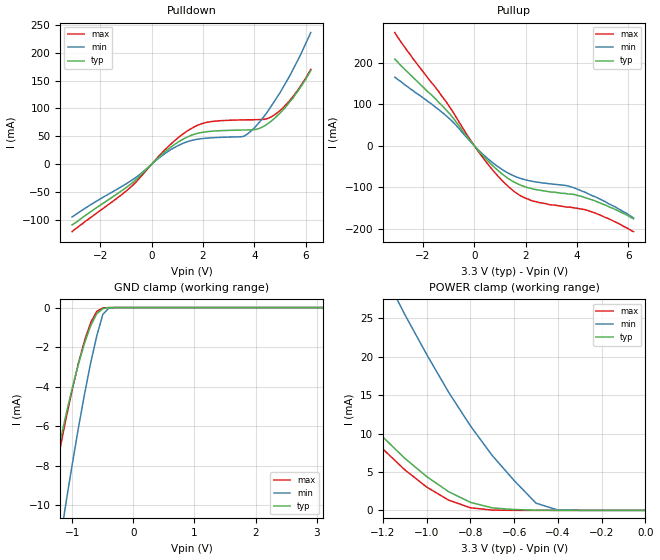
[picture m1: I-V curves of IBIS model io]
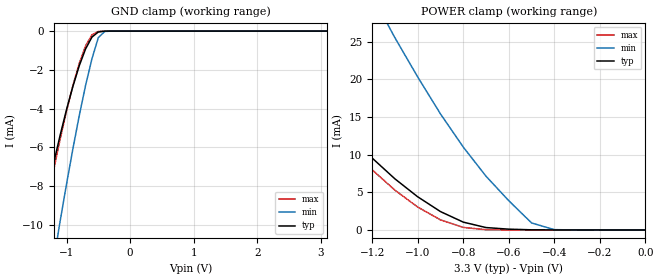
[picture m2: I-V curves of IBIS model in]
[IBIS Ver]   1.1
[File name]   m63733a.ibs
[File Rev]   1.0
[Date]   7/28/98
[Source]   This file originated at Motorola Fast SRAM.
[Notes]
 1. This I/O model good for MCM63733A 128Kx32 4Mb BurstRAM "F" and "P" versions (TQFP).
[Disclaimer]   Data is for modeling purposes only and is not guaranteed
[Component]   128Kx32 4Mb BurstRAM
[Manufacturer] Motorola
[Package]
|  RLC Data is subject to change after further study of package
|		typ		min		max
R_pkg		200m		150m		250m
L_pkg		5.5nH		4nH		7nH
C_pkg		2pF		1.5pF		2.5pF
[Pin]		signal_name	model_name	R_pin		L_pin		C_pin
1		NC		NC		NA		NA		NA
2		DCc		io		NA		NA		NA
3		DCc		io		NA		NA		NA
4		VDDQ		POWER		NA		NA		NA
5		VSS		GND		NA		NA		NA
6		DCc		io		NA		NA		NA
7		DCc		io		NA		NA		NA
8		DQc		io		NA		NA		NA
9		DQc		io		NA		NA		NA
10		VSS		GND		NA		NA		NA
11		VDDQ		POWER		NA		NA		NA
12		DQc		io		NA		NA		NA
13		DQc		io		NA		NA		NA
14		NC		NC		NA		NA		NA
15		VDD		POWER		NA		NA		NA
16		NC		NC		NA		NA		NA
17		VSS		GND		NA		NA		NA
18		DQd		io		NA		NA		NA
19		DQd	 	io		NA		NA		NA
20		VDDQ		POWER		NA		NA		NA
21		VSS		GND		NA		NA		NA
22		DQd		io		NA		NA		NA
23		DQd		io		NA		NA		NA
24		DQd		io		NA		NA		NA
25		DCd		io		NA		NA		NA
26		VSS		GND		NA		NA		NA
27		VDDQ		POWER		NA		NA		NA
28		DCd		io		NA		NA		NA
29		DCd		io		NA		NA		NA
30		NC		NC		NA		NA		NA
31		LBO#		NC		NA		NA		NA
32		SA		in		NA		NA		NA
33		SA		in		NA		NA		NA
34		SA		in		NA		NA		NA
35		SA		in		NA		NA		NA
36		SA1		in		NA		NA		NA
37		SA0		in		NA		NA		NA
38		NC		NC		NA		NA		NA
39		NC		NC		NA		NA		NA
40		VSS		GND		NA		NA		NA
41		VDD		POWER		NA		NA		NA
42		NC		NC		NA		NA		NA
43		NC		NC		NA		NA		NA
44		SA		in		NA		NA		NA
45		SA		in		NA		NA		NA
46		SA		in		NA		NA		NA
47		SA		in		NA		NA		NA
48		SA		in		NA		NA		NA
49		SA		in		NA		NA		NA
50		SA		in		NA		NA		NA
51		NC		NC		NA		NA		NA
52		DQa		io		NA		NA		NA
53		DQa		io		NA		NA		NA
54		VDDQ		POWER		NA		NA		NA
55		VSS		GND		NA		NA		NA
56		DQa		io		NA		NA		NA
57		DQa		io		NA		NA		NA
58		DQa		io		NA		NA		NA
59		DQa		io		NA		NA		NA
60		VSS		GND		NA		NA		NA
61		VDDQ		POWER		NA		NA		NA
62		DQa		io		NA		NA		NA
63		DQa		io		NA		NA		NA
64		ZZ		NC		NA		NA		NA
65		VDD		POWER		NA		NA		NA
66		NC		NC		NA		NA		NA
67		VSS		GND		NA		NA		NA
68		DQb		io		NA		NA		NA
69		DQb		io		NA		NA		NA
70		VDDQ		POWER		NA		NA		NA
71		VSS		GND		NA		NA		NA
72		DQb		io		NA		NA		NA
73		DQb		io		NA		NA		NA
74		DQb		io		NA		NA		NA
75		DQb		io		NA		NA		NA
76		VSS		GND		NA		NA		NA
77		VDDQ		POWER		NA		NA		NA
78		DQb		io		NA		NA		NA
79		DQb		io		NA		NA		NA
80		NC		NC		NA		NA		NA
81		SA		in		NA		NA		NA
82		SA		in		NA		NA		NA
83		ADV		in		NA		NA		NA
84		ADSP		in		NA		NA		NA
85		ADSC		in		NA		NA		NA
86		G#		in		NA		NA		NA
87		SW#		in		NA		NA		NA
88		SGW#		in		NA		NA		NA
89		K		in		NA		NA		NA
90		VSS		GND		NA		NA		NA
91		VDD		POWER		NA		NA		NA
92		SE3#		in		NA		NA		NA
93		SBA#		in		NA		NA		NA
94		SBB#		in		NA		NA		NA
95		SBC#		NC		NA		NA		NA
96		SBD#		NC		NA		NA		NA
97		SE2		in		NA		NA		NA
98		SE1#		in		NA		NA		NA
99		SA		in		NA		NA		NA
100		SA		in		NA		NA		NA
| Models and submodels in the file (2): io (I/O), in (Input)
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| BI-DIRECTIONAL I/O MODEL
[Model]   io
Model_type  I/O
Polarity   Non-Inverting
Enable   Active-Low
|signals  DQa, DQb, DQc, DQd
|Variable   typ   min   max
C_comp   7pF   NA   8pF
|Variable   typ   min   max
[Voltage range]   3.3   3.1  3.6
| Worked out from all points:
|   slope of the pulldown table from 0 to 0.495 V, typ, clamps not added: 23.3 ohm
|   slope of the pullup table from 0 to 0.495 V, typ, clamps not added: 14.4 ohm
|   GND clamp passes 1 mA (typ) near -0.71 V on its own axis
|   POWER clamp passes 1 mA (typ) near -0.79 V on its own axis
|Temp used   50C   100C   0C
|Variable   typ   min   max
|NOTE: All V/I tables should have at least 3 entries.
|   0.0 volts, 2*supply_voltage and -supply_voltage
[Pulldown]
|Volt	Typical		Minimum		Maximum
-3.1V     -109mA     -94.7mA    -121mA
-900mV    -38.8mA    -32.6mA    -44.6mA
500mV     21.4mA     18.4mA     25mA
1.4V      48.9mA     40.4mA     59.8mA
2.2V      58.5mA     46.8mA     75.4mA
3.5V      61.2mA     49.2mA     79.3mA
3.8V      61.4mA     56.5mA     79.6mA
4.3V      66.3mA     81mA       80mA
4.6V      75.1mA     99.8mA     83.5mA
4.9V      87mA       121mA      92.3mA
5.4V      113mA      160mA      115mA
6.2V      168mA      236mA      170mA
[Pullup]
|Volt	Typical		Minimum		Maximum
-3.1V     208mA      165mA      272mA
-2.4V     165mA      133mA      210mA
-1.1V     86.2mA     72.2mA     106mA
-200mV    15.4mA     13.3mA     18.3mA
300mV     -21.4mA    -18.4mA    -25.8mA
900mV     -58.1mA    -49.2mA    -71.3mA
1.4V      -81.6mA    -68.2mA    -102mA
1.8V      -94.4mA    -78.2mA    -120mA
2.3V      -104mA     -85.6mA    -133mA
3.9V      -117mA     -101mA     -149mA
4.7V      -132mA     -122mA     -161mA
6.2V      -175mA     -173mA     -206mA
[GND_clamp]
|Volt	Typical		Minimum		Maximum
-3.1V     -45.8mA    -60.1mA    -49.3mA
-1.5V     -11.5mA    -18.1mA    -12.3mA
-1.4V     -9.83mA    -15.9mA    -10.5mA
-1.2V     -6.78mA    -11.8mA    -7.13mA
-1.1V     -5.37mA    -9.8mA     -5.57mA
-900mV    -2.86mA    -6.08mA    -2.81mA
-800mV    -1.79mA    -4.37mA    -1.67mA
-700mV    -918uA     -2.8mA     -759uA
-600mV    -310uA     -1.43mA    -192uA
-500mV    -48.2uA    -340uA     -17.7uA
-300mV    -165nA     -1.28uA    -19.6nA
3.1V      425pA      626pA      394pA
[POWER_clamp]
|Volt	Typical		Minimum		Maximum
-3.1V     105mA      173mA      110mA
-1.7V     27.7mA     62.5mA     26.7mA
-1.6V     23.6mA     55.8mA     22.4mA
-1.4V     16mA       43mA       14.5mA
-1.2V     9.54mA     31.1mA     7.98mA
-1.1V     6.78mA     25.5mA     5.28mA
-900mV    2.44mA     15.4mA     1.34mA
-800mV    1.04mA     11mA       338uA
-700mV    319uA      7.13mA     33.9uA
-500mV    20.9uA     933uA      150nA
-400mV    578nA      41.7uA     2.74nA
0V        469pA      626pA      504pA
[Ramp]
|Variable   typ   min	max
dV/dt_r  1.50/0.33n	NA	NA
dV/dt_f  1.29/0.13n	NA	NA
| STANDARD INPUT MODEL
[Model]   in
Model_type  Input
Polarity   Non-Inverting
|signals  ADSP#, ADSC#, ADV#, G#, K, SA, SBx#, SE1#, SE2, SE3#, SGW#, SW#
|Variable   typ   min   max
C_comp   4pF   NA   5pF
|Variable   typ   min   max
[Voltage range]   3.3   3.1  3.6
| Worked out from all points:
|   GND clamp passes 1 mA (typ) near -0.71 V on its own axis
|   POWER clamp passes 1 mA (typ) near -0.79 V on its own axis
|Temp used   50C   100C   0C
[GND_clamp]
|Volt	Typical		Minimum		Maximum
-3.1V     -45.8mA    -60.1mA    -49.3mA
-1.5V     -11.5mA    -18.1mA    -12.3mA
-1.4V     -9.83mA    -15.9mA    -10.5mA
-1.2V     -6.78mA    -11.8mA    -7.13mA
-1.1V     -5.37mA    -9.8mA     -5.57mA
-900mV    -2.86mA    -6.08mA    -2.81mA
-800mV    -1.79mA    -4.37mA    -1.67mA
-700mV    -918uA     -2.8mA     -759uA
-600mV    -310uA     -1.43mA    -192uA
-500mV    -48.2uA    -340uA     -17.7uA
-300mV    -165nA     -1.28uA    -19.6nA
3.1V      425pA      626pA      394pA
[POWER_clamp]
|Volt	Typical		Minimum		Maximum
-3.1V     105mA      173mA      110mA
-1.7V     27.7mA     62.5mA     26.7mA
-1.6V     23.6mA     55.8mA     22.4mA
-1.4V     16mA       43mA       14.5mA
-1.2V     9.54mA     31.1mA     7.98mA
-1.1V     6.78mA     25.5mA     5.28mA
-900mV    2.44mA     15.4mA     1.34mA
-800mV    1.04mA     11mA       338uA
-700mV    319uA      7.13mA     33.9uA
-500mV    20.9uA     933uA      150nA
-400mV    578nA      41.7uA     2.74nA
0V        469pA      626pA      504pA
